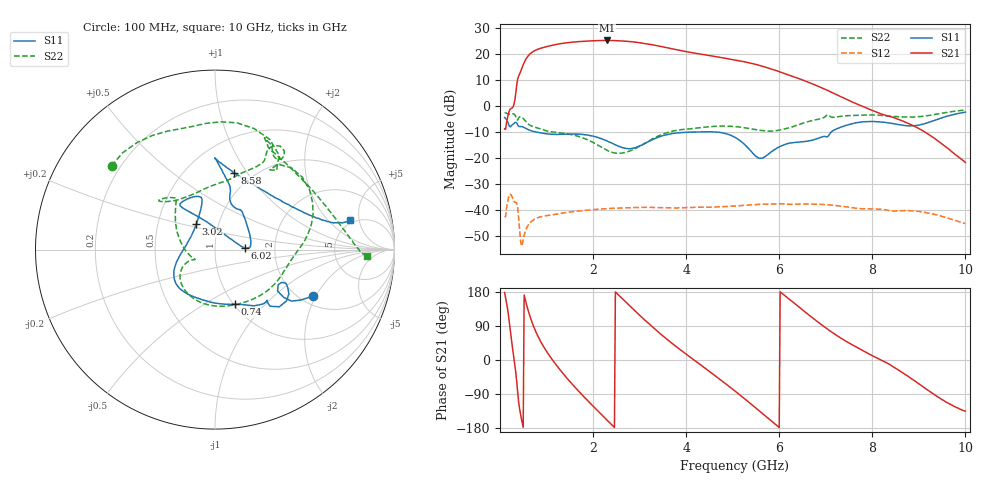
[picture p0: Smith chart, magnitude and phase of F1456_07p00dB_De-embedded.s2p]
! Integrated Device Technology
! Corporate Headquarters
! 6024 Silver Creek Valley Road
! San Jose, CA 95138  USA
! Phone:  1-408-284-8200
! Toll Free:  1-800-223-1366
! Webpage:  http://www.idt.com/
! Timing and RF Division
! 515 Groton Road, Suite 102
! Westford, MA 01886-6024
! Device:  F1456
! Description: 6-bit 0.5 dB Transmit Variable Gain Amplifier
! Frequency:  2100.0 -  2950.00 MHz
! Package:  6x6 mm Thin QFN Plastic Package: 28 pin
! State:  14
! Atten State:  7.0 dB
! Voltage:  +5.00 Volts
! Current:  217.047 mA
! Data:  The device was measured on a the F1455 evaluation board which has
!  individual transmission lines to the RF pins.  Data was collected
!  using a calibrated network analyzer.  The evaluation board was
!  de-embedded using a TRL calibration technique.
!  The reference plane is the edge of the package pin.
!  Pin  1 = CSb
!  Pin  2 = DATA
!  Pin  3 = CLK
!  Pin  4 = RSET
!  Pin  5 = GND
!  Pin  6 = RFIN  = Port 1
!  Pin  7 = GND
!  Pin  8 = NC
!  Pin  9 = NC
!  Pin 10 = NC
!  Pin 11 = NC
!  Pin 12 = NC
!  Pin 13 = NC
!  Pin 14 = /STBY
!  Pin 15 = GND
!  Pin 16 = RFOUT  = Port 2
!  Pin 17 = GND
!  Pin 18 = NC
!  Pin 19 = NC
!  Pin 20 = NC
!  Pin 21 = GND
!  Pin 22 = NC
!  Pin 23 = GND
!  Pin 24 = NC
!  Pin 25 = NC
!  Pin 26 = NC
!  Pin 27 = GND
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# GHz S dB R 50
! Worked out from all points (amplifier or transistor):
!   496 points, 100 MHz to 10 GHz, reference 50 ohm
!   highest |S21| = 25.3 dB at 2.3 GHz (marker M1)
!   |S21| within 3 dB of that: 876.8 MHz to 3.647 GHz (2.77 GHz wide, 122 % of centre)
!   unconditionally stable (mu >= 1): start of sweep to end of sweep
!   at 1.74 GHz: K = 2.64, MAG = 25.5 dB, |S12| = -40.2 dB
!   at 5.06 GHz: K = 4.28, MAG = 18.8 dB, |S12| = -38.3 dB
!   at 10 GHz: K = 127.18, MAG = -12.3 dB, |S12| = -45.2 dB
!   S11 on the Smith chart (normalised r, x): 100 MHz: 2.33, -1.91; 740 MHz: 1.01, -0.69; 3.02 GHz: 0.78, +0.23; 6.02 GHz: 1.40, +0.03; 8.58 GHz: 0.82, +0.87; 10 GHz: 4.63, +3.75
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0.1  -4.35 -25.3  -8.69 178.2  -42.37 44.6  -2.61 141.0
0.34  -6.19 -35.7  5.02 -32.5  -37.02 -147.2  -3.93 55.9
0.42  -7.81 -44.0  12.30 -127.6  -46.97 136.6  -4.10 46.9
0.56  -8.58 -56.9  18.18 151.5  -47.32 -174.2  -5.94 6.0
0.74  -9.78 -70.0  21.34 83.5  -43.51 135.7  -8.00 -20.4
0.96  -10.51 -88.9  22.75 30.8  -42.22 92.7  -9.28 -55.2
1.2  -10.84 -107.9  23.76 -11.6  -41.55 64.5  -10.03 -88.3
1.5  -10.69 -126.5  24.55 -56.6  -40.70 38.5  -10.79 -121.6
1.76  -10.82 -139.3  24.95 -91.4  -40.17 20.2  -12.04 -141.1
2.02  -11.60 -150.6  25.21 -124.2  -39.76 4.2  -14.12 -152.8
2.3  -13.34 -165.1  25.32 -158.6  -39.40 -12.0  -16.95 -155.8
2.62  -15.89 169.6  25.14 162.8  -39.12 -29.6  -18.05 -154.6
3.02  -15.11 126.7  24.40 115.8  -38.93 -50.7  -15.17 177.0
3.4  -11.94 107.4  23.22 74.0  -38.98 -69.4  -11.49 145.1
4.1  -9.95 113.0  20.71 6.5  -38.97 -98.4  -8.66 128.5
4.6  -9.87 127.1  19.20 -39.4  -38.79 -119.4  -7.74 136.5
5.06  -12.06 123.7  17.78 -82.9  -38.33 -138.7  -7.83 138.6
6.02  -15.46 3.1  13.19 179.8  -37.54 169.3  -9.12 95.9
6.7  -13.12 34.9  8.70 112.8  -37.63 128.9  -5.55 62.7
8.36  -6.43 85.0  -3.84 -10.9  -40.19 53.0  -3.83 62.6
8.58  -7.11 75.8  -5.18 -28.0  -40.23 47.5  -4.03 56.7
10  -2.25 12.3  -21.65 -134.9  -45.17 -30.7  -1.46 -2.5
